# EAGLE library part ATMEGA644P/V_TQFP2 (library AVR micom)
ATMEGA644P TQFP pacage AVR micon series. producted by ATMEL.Co
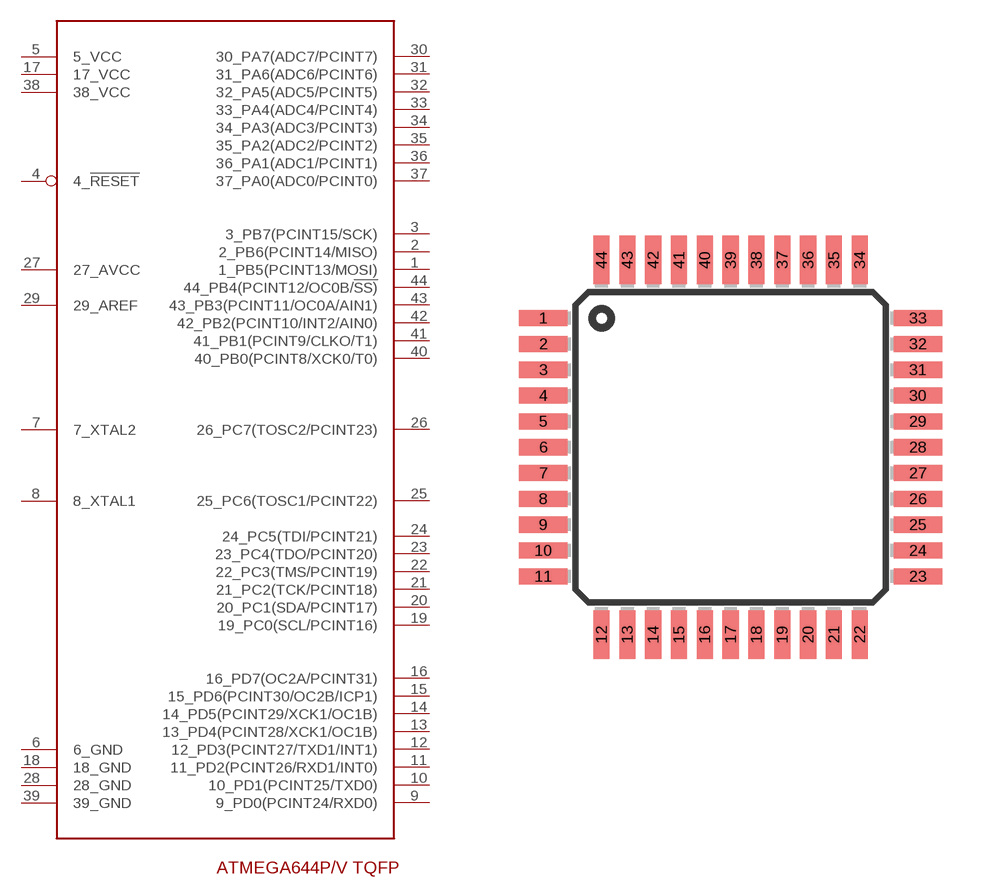
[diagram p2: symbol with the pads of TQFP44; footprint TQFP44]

Designator prefix U

## ATMEGA644P/V_TQFP2  [TQFP44]
1  1_PB5(PCINT13/MOSI)
2  2_PB6(PCINT14/MISO)
3  3_PB7(PCINT15/SCK)
4  4_!RESET
5  5_VCC
6  6_GND
7  7_XTAL2
8  8_XTAL1
9  9_PD0(PCINT24/RXD0)
10  10_PD1(PCINT25/TXD0)
11  11_PD2(PCINT26/RXD1/INT0)
12  12_PD3(PCINT27/TXD1/INT1)
13  13_PD4(PCINT28/XCK1/OC1B)
14  14_PD5(PCINT29/XCK1/OC1B)
15  15_PD6(PCINT30/OC2B/ICP1)
16  16_PD7(OC2A/PCINT31)
17  17_VCC
18  18_GND
19  19_PC0(SCL/PCINT16)
20  20_PC1(SDA/PCINT17)
21  21_PC2(TCK/PCINT18)
22  22_PC3(TMS/PCINT19)
23  23_PC4(TDO/PCINT20)
24  24_PC5(TDI/PCINT21)
25  25_PC6(TOSC1/PCINT22)
26  26_PC7(TOSC2/PCINT23)
27  27_AVCC
28  28_GND
29  29_AREF
30  30_PA7(ADC7/PCINT7)
31  31_PA6(ADC6/PCINT6)
32  32_PA5(ADC5/PCINT5)
33  33_PA4(ADC4/PCINT4)
34  34_PA3(ADC3/PCINT3)
35  35_PA2(ADC2/PCINT2)
36  36_PA1(ADC1/PCINT1)
37  37_PA0(ADC0/PCINT0)
38  38_VCC
39  39_GND
40  40_PB0(PCINT8/XCK0/T0)
41  41_PB1(PCINT9/CLKO/T1)
42  42_PB2(PCINT10/INT2/AIN0)
43  43_PB3(PCINT11/OC0A/AIN1)
44  44_PB4(PCINT12/OC0B/!SS)

## Footprint TQFP44 (pad centres in mm)
Thin Plasic Quad Flat Package
smd 1.5 x 0.5: 1 -5.8,4; 2 -5.8,3.2; 3 -5.8,2.4; 4 -5.8,1.6; 5 -5.8,0.8; 6 -5.8,0; 7 -5.8,-0.8; 8 -5.8,-1.6; 9 -5.8,-2.4; 10 -5.8,-3.2; 11 -5.8,-4; 23 5.8,-4; 24 5.8,-3.2; 25 5.8,-2.4; 26 5.8,-1.6; 27 5.8,-0.8; 28 5.8,0; 29 5.8,0.8; 30 5.8,1.6; 31 5.8,2.4; 32 5.8,3.2; 33 5.8,4
smd 0.5 x 1.5: 12 -4,-5.8; 13 -3.2,-5.8; 14 -2.4,-5.8; 15 -1.6,-5.8; 16 -0.8,-5.8; 17 0,-5.8; 18 0.8,-5.8; 19 1.6,-5.8; 20 2.4,-5.8; 21 3.2,-5.8; 22 4,-5.8; 34 4,5.8; 35 3.2,5.8; 36 2.4,5.8; 37 1.6,5.8; 38 0.8,5.8; 39 0,5.8; 40 -0.8,5.8; 41 -1.6,5.8; 42 -2.4,5.8; 43 -3.2,5.8; 44 -4,5.8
